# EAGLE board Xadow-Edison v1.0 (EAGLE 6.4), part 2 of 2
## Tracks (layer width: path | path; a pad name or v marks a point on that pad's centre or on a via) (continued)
SPI_MOSI/D11  (via drill 0.1 pad 0.25 layers 1-2, 0.3 pad 0.64) (continued)
  Route2 0.102: v17.14,36.32 17.14,36.96 17.4,37.21 18.16,37.21 18.41,36.96 18.41,36.07 18.16,35.81 18.16,31.75 17.14,30.73 17.14,28.96 18.41,27.69 18.41,25.53 17.53,24.64 17.53,23.88 18.16,23.24 18.16,21.21 20.19,19.18 20.19,17.65 19.56,17.02 19.56,12.95 18.16,11.56 18.16,11.3 18.41,11.05 18.41,10.16 18.16,9.91 18.16,9.27 18.41,9.02 18.41,8.51 18.16,8.26 18.16,6.73 v18.01,6.58
  Bottom 0.102: v10.99,4.7 12.89,4.7 13.91,3.68 13.91,1.97 14.22,1.65 15.11,1.65 15.37,1.91 v15.37,2.29
SYS  (via drill 0.3 pad 0.64)
  Top 0.254: U19.15 v26.42,33.33 v26.42,33.34 | U19.1 25.2,32.21 v25.15,32.26 | v27.56,28.45 27.56,28 R31.1
  Route2 0.61: v25.15,32.26 25.34,32.26 v26.42,33.34
  Bottom 0.254: v25.15,32.26 25.15,28.19 25.65,27.69 26.8,27.69 v27.56,28.45
  Bottom 0.61: v25.15,32.26 24.38,32.26 22.99,30.86 20.45,30.86 19.74,30.15 v19.74,29.62
  pour Top (isolate 0.254, no thermals): 22.22,27.81 21.46,27.81 21.21,28.07 21.21,29.08 20.95,29.34 19.05,29.34 18.8,29.59 18.8,30.61 18.92,30.73 21.84,30.73 21.97,30.61 21.97,29.84 22.1,29.72 22.48,29.72 22.61,29.59 22.61,27.94 22.48,27.81
UART1_CTS  (via drill 0.1 pad 0.25 layers 1-2, 0.3 pad 0.64)
  Top 0.102: U26.4 6.67,10.8 v6.67,10.79 | J2.17 4.08,16.75 v4.06,16.76 | R63.1 v1.46,7.11
  Route2 0.102: v4.06,16.76 4.06,16.38 4.83,15.62 4.83,14.22 4.57,13.97 4.57,13.46 6.67,11.37 v6.67,10.79 6.67,10.48 6.35,10.16 4.06,10.16 1.46,7.56 v1.46,7.11
UART1_RTS  (via drill 0.1 pad 0.25 layers 1-2, 0.3 pad 0.64)
  Top 0.102: U27.4 8.76,8.25 8.38,7.87 v8,7.87 | J2.18 6.47,16.25 6.93,16.71 v7.75,16.71 | R62.1 v1.14,5.33
  Route2 0.102: v7.75,16.71 7.75,16.51 8.95,15.3 9.33,15.3 9.53,15.11 9.53,14.61 8.89,13.97 8.45,13.97 7.81,13.34 7.81,12.08 7.37,11.63 7.37,10.41 6.98,10.03 6.98,8.64 7.75,7.87 v8,7.87 8.26,7.87 8.76,7.37 8.76,5.57 7.39,4.19 2.29,4.19 v1.14,5.33
UART1_RX  (via drill 0.1 pad 0.25 layers 1-2, 0.3 pad 0.64)
  Top 0.102: J3.2 12.88,3.03 v12.83,2.98 | J4.11 12.88,36.04 v12.8,36.12 | U9.4 14.6,10.54 v14.35,10.29 | R59.1 1.84,8.95 2.33,9.44 3.51,9.44 3.94,9.02 v3.94,8.51
  Route2 0.102: v12.83,2.98 12.83,6.1 13.83,7.1 13.83,8.14 13.59,8.38 13.59,9.53 v14.35,10.29 14.48,10.41 14.48,11.81 13.97,12.32 13.97,13.97 13.84,14.1 13.84,18.92 13.34,19.43 13.34,21.72 13.72,22.1 13.97,22.1 14.48,22.61 14.48,23.37 14.26,23.58 14.26,24.68 14.73,25.15 14.73,28.57 15.37,29.21 15.37,30.35 14.86,30.86 13.97,30.86 13.34,31.5 13.34,35.59 v12.8,36.12
  Bottom 0.102: v12.83,2.98 12.19,3.62 10.6,3.62 9.02,2.03 7.11,2.03 4.19,4.95 4.19,8.26 v3.94,8.51 3.94,9.27 P2.00
UART1_TX  (via drill 0.1 pad 0.25 layers 1-2, 0.3 pad 0.64)
  Top 0.102: U8.4 v12.82,10.8 v12.83,10.79 | J3.1 12.38,3.8 v11.62,3.05 | J4.12 12.38,34.1 v12.45,34.04 | R60.1 1.4,8 1.14,8.26 1.14,9.3 v1.52,9.68
  Route2 0.102: v11.62,3.05 11.81,3.24 11.81,7.62 12.08,7.89 12.08,8.88 11.94,9.02 11.94,9.91 v12.83,10.79 12.83,11.68 13.21,12.06 13.21,13.59 13.08,13.72 13.08,18.54 12.57,19.05 12.57,22.61 13.34,23.37 13.34,24.51 14.22,25.4 14.22,28.83 14.86,29.46 14.86,30.1 14.61,30.35 13.72,30.35 12.83,31.24 12.83,33.66 v12.45,34.04
  Bottom 0.102: v1.52,9.68 2.01,9.68 P1.00 2.29,8.51 3.43,7.37 3.43,2.79 4.44,1.78 9.14,1.78 10.41,3.05 v11.62,3.05
USB_DN  (via drill 0.3 pad 0.64)
  Top 0.102: J9.10 26.63,21.43 v26.8,21.27
  Bottom 0.102: J1.18 5.81,19.53 6.73,20.45 7.87,20.45 8.51,19.81 14.99,19.81 15.75,20.57 24,20.57 arc90 24.26,20.83 24.26,20.95 arc-90 24.51,21.21 arc-90 24.77,20.95 24.77,20.83 arc90 25.02,20.57 arc90 25.27,20.83 25.27,20.95 arc-90 25.53,21.21 arc-90 25.78,20.95 25.78,20.83 arc90 26.04,20.57 26.49,20.57 arc45 26.58,20.61 26.76,20.79 arc45 26.8,20.88 v26.8,21.27
USB_DP  (via drill 0.3 pad 0.64)
  Top 0.102: J9.11 26.63,21.93 v26.8,22.1
  Bottom 0.102: J1.16 5.79,19.13 6.86,20.19 7.75,20.19 8.38,19.56 15.11,19.56 15.88,20.32 26.62,20.32 arc45 26.71,20.36 27.3,20.95 arc45 27.34,21.04 27.34,21.5 arc45 27.3,21.59 v26.8,22.1
USB_ID  (via drill 0.3 pad 0.64)
  Top 0.102: J9.3 26.52,17.93 26.96,17.49 26.96,15.91 v26.48,15.43
  Bottom 0.102: J1.3 2.83,16.73 3.05,16.51 3.05,15.62 3.3,15.37 5.21,15.37 5.84,14.73 5.84,14.1 6.22,13.72 10.92,13.72 11.18,13.97 22.61,13.97 22.99,14.35 24.38,14.35 24.77,14.73 24.77,15.62 25.02,15.88 26.04,15.88 v26.48,15.43
USB_VBUS  (via drill 0.3 pad 0.64)
  Top 0.305: J9.8 24.4,20.43 23.88,20.95 23.88,22.92 v23.81,22.99
  Bottom 0.203: J1.20 5.58,19.93 5.59,19.94
  Bottom 0.305: 5.59,19.94 7.37,21.72 14.1,21.72 14.99,22.61 18.99,22.61 19.62,23.24 23.56,23.24 v23.81,22.99
VCC_1V8  (via drill 0.3 pad 0.64)
  Top 0.102: U26.1
  Top 0.203: 27.37,4.25 v27.3,4.32 27.62,4 R39.1
  Top 0.254: U24.1 10.03,12.06 10.03,12.57 | U8.1 11.81,12.19 11.81,12.83 | U9.1 13.72,12.19 13.72,12.7 | U22.1 17.02,12.06 17.02,12.7 | 13.72,12.7 13.72,13.08 | 13.72,12.7 13.97,12.95 | 13.72,12.7 13.46,12.95 | U5.1 18.62,12.37 v18.62,13.16 | U25.1 13.34,8.64 13.34,9.65 | U27.1 v8.26,10.18 | U6.1 18.67,8.89 v18.67,9.65 | U3.1 16.89,8.76 16.89,9.27 | 16.89,9.27 16.89,9.65 | 16.89,9.27 17.14,9.53 | 16.89,9.27 16.64,9.53 | U11.1 14.86,8.89 14.86,9.27 | 14.86,9.27 14.86,9.65 | 14.86,9.27 14.61,9.53 | 14.86,9.27 15.11,9.53 | C4.1 | U26.1 6.1,11.94 v6.1,12.87 | U17.21 v19.43,18.67 19.43,19.3 19.06,19.67 U17.23 | U7.1 11.43,9.86 | 11.43,9.9 11.43,10.18 11.43,10.19 | 11.43,9.86 11.43,9.9 | 11.43,9.9 11.3,10.03 | 11.43,9.86 11.44,9.86 11.61,10.03 | U23.1 8.26,13.01 R47.2 | U10.2 8.99,26.87 v9.14,27.03 | 11.81,12.83 11.81,13.18 | 11.81,12.83 11.56,13.08 | 11.81,12.83 12.07,13.08 | 17.02,12.7 17.02,13.08 | 17.02,12.7 16.76,12.95 | 17.02,12.7 17.27,12.95 | R35.2 v28.96,33.53 | 10.03,12.65 10.03,12.93 | 10.03,12.57 10.03,12.65 | 10.03,12.65 10.31,12.93 | 10.03,12.57 9.78,12.83
  Top 0.305: C4.1 U2.21 | U15.8 12.02,24.25 v11.91,24.14 | U16.8 10.02,34.41 v10.11,34.49 | U14.8 11.8,21.32 v11.56,21.08 | U12.8 11.95,18.53 v11.94,18.54
  Top 0.406: U13.5 v6.24,30.72 5.73,31.23 4.94,31.23 4.57,30.86 4.57,30.23 3.85,29.5 R14.2
  Top 0.508: 16.13,13.08 15.49,13.08 | 15.49,13.08 13.72,13.08 12.8,13.08 v12.7,13.18 | v18.67,9.65 16.89,9.65 14.86,9.65 13.34,9.65 12.8,10.19 11.43,10.19 9.78,10.19 | v8.26,10.18 v8.26,10.19 9.78,10.19 | C4.1 C3.1 14.99,23.75 15.27,24.03 v15.32,24.03 | R46.2 15.88,12.7 | 15.88,12.7 15.88,12.83 16.13,13.08 | 15.88,12.7 15.49,13.08 | R30.2 10.08,9.88 | 10.08,9.88 9.78,10.19 | 10.08,9.88 10.34,10.13 | R42.2 12.83,13.31 v12.7,13.18 | R36.2 7.05,38.16 7.05,37.96 v6.86,37.77 6.78,37.85 Q4.1 | Q3.1 6.1,35.56 6.54,36.01 R2.2 | R15.1 v11.15,26.29 | 11.02,13.18 Q2.1 | v12.7,13.18 11.81,13.18 11.02,13.18 | 16.13,13.08 17.02,13.08 17.14,13.08 17.21,13.14 17.27,13.21 Q1.1 | C14.1 9.42,27.3 v9.14,27.03 | R40.2 18.41,13.41 18.67,13.16 18.54,13.16 | R47.2 9.27,13.08 9.42,12.93 v9.53,12.93 10.03,12.93 10.13,12.93 10.39,13.18 11.02,13.18
  Top 0.61: v19.43,18.67 19.88,18.67 C17.1 | v10.11,34.49 10.11,34.85 9.78,35.18 8.38,35.18 8.13,35.43 | 8.13,35.43 v8.13,35.37 | v18.62,13.16 18.54,13.16 17.22,13.16 17.21,13.14 | R2.2 7.56,36.01 8.13,35.43 | v7.19,19.1 7.3,19.21 C33.1 C34.1
  Route2 0.203: v22.99,38.73 22.73,38.73 22.61,38.61
  Route2 0.61: v12.7,13.18 12.57,13.31 12.57,17.91 v11.94,18.54 11.94,20.7 v11.56,21.08 | v15.32,24.03 15.6,24.03 17.4,22.23 17.4,20.7 v19.43,18.67 19.43,18.03 18.62,17.22 v18.62,13.16 | v8.13,35.37 8.13,38.23 | 8.51,38.61 7.75,38.61 | 8.13,38.23 7.75,38.61 | 8.13,38.23 8.51,38.61 | v6.24,30.72 7.05,31.53 8.47,31.53 9.91,30.1 9.91,29.34 9.4,28.83 9.4,27.28 v9.14,27.03 | v6.86,37.77 6.86,38.23 7.24,38.61 7.75,38.61 | v28.96,33.53 27.56,34.92 27.56,35.69 24.64,38.61 22.61,38.61 8.51,38.61
  Bottom 0.203: J1.12 6.81,18.33 | 6.81,18.33 7.41,18.33 7.46,18.38 | v27.3,4.32 27.81,4.32 28.32,4.83 28.32,5.71 28.83,6.22 28.83,9.14 28.45,9.53 28.45,10.92 29.63,12.11 29.63,16.21 28.51,17.34 26.8,17.34 25.53,18.61 19.49,18.61 v19.43,18.67 | 6.81,18.33 6.81,18.37 7.11,18.67 | 1.8V.T v22.99,38.73
  Bottom 0.508: 9.17,27.05 v9.14,27.03 | v6.1,12.87 6.13,12.87 6.22,12.95 9.5,12.95 v9.53,12.93
  Bottom 0.61: v18.67,9.65 18.67,10.03 20.57,11.94 20.57,12.7 20.12,13.16 v18.62,13.16 | v15.32,24.03 13.08,24.03 | 13.08,24.03 12.57,24.03 | 12.57,24.03 12.03,24.03 v11.91,24.14 | 13.08,24.64 13.08,24.51 | 13.08,24.51 13.08,24.03 | 13.08,24.51 13.06,24.51 12.57,24.03 | 13.08,24.64 13.59,24.13 | v8.13,35.37 8.06,35.37 6.73,34.04 6.73,31.21 v6.24,30.72 | 13.08,24.64 13.08,25.53 12.32,26.29 v11.15,26.29 9.88,26.29 v9.14,27.03 | v7.19,19.1 7.19,18.66 7.46,18.38 7.75,18.1 11.49,18.1 v11.94,18.54
VCC_3V3  (via drill 0.3 pad 0.64)
  Top 0.203: R38.1 27.88,6.22 v28.19,6.54
  Top 0.254: U7.6 v12.41,9.39 v12.42,9.4 | U11.6 v15.87,8.89 v15.88,8.89 | U3.6 v17.78,8.89 | U25.6 v14.09,8.89 v14.1,8.89 | U24.6 v10.79,12.31 v10.79,12.32 | U22.6 v17.78,12.31 v17.78,12.32 | U27.6 9.17,9.52 v9.24,9.45 | U18.21 6.47,8.01 v6.1,8.38 | U9.6 14.6,12.19 v14.73,12.31 | U8.6 v12.7,12.31 v12.7,12.32 | U5.6 v19.68,12.26 v19.68,12.27 | U6.6 19.68,8.77 v19.56,8.89 | U18.18 v8.22,7.23 v8.23,7.24 | U4.21 21.97,10.03 21.78,9.84 C16.1 | U26.6 v6.73,12.21 v6.73,12.22 | U23.6 8.76,11.93 v9.02,12.19
  Top 0.305: J3.5 14.38,4.04 14.68,3.73 v15.27,3.73 15.54,3.73 15.88,4.07 J3.8 | v6.71,17.6 6.48,17.83 6.48,18.92 6.15,19.25 J2.12 | 15.62,33.78 14.61,33.78 14.38,34.01 J4.8 14.38,36.22 v15.11,36.96 | 15.62,33.78 15.88,33.78 | 15.88,33.78 16.13,33.78 | 16.13,33.78 v19.18,33.78 | 15.88,33.78 | J4.5 15.88,34.03 | 15.88,34.03 16.13,33.78 | 15.88,34.03 15.87,34.03 15.62,33.78
  Top 0.508: R41.2 13.97,14.92 v14.35,15.3 | C16.1 21.21,9.35 v21.18,9.32 21.21,9.3 R44.2 | R67.2 R3.2 3.87,37.02 v3.94,37.08 | C7.1 20.07,22.73 v19.84,22.5 19.46,22.5 19.18,22.23 R7.2
  Top 0.61: C32.1 C31.1 7.04,17.27 v6.71,17.6 | R43.2 6.6,14.1 v6.41,14.29 | v19.68,12.26 19.68,12.66 20.99,13.97 21.84,13.97 22.29,14.41 R45.2 22.73,14.99 v22.48,15.24
  Route2 0.203: v28.19,6.54 28.19,9.98 26.49,11.68 23.88,11.68 23.43,12.13 23.43,14.29 v22.48,15.24
  Route2 0.508: v14.35,15.3 14.35,14.73 14.73,14.35 v14.73,12.31 | v15.11,36.96 15.11,37.08 14.5,37.7 11.54,37.7 v10.16,36.32
  Route2 0.61: v6.71,17.6 6.35,17.25 6.35,14.35 v6.41,14.29 6.86,13.84 6.86,12.34 v6.73,12.22 | v19.56,8.89 20.07,8.89 20.5,9.32 v21.18,9.32 | v19.18,33.78 19.18,31.24 18.92,30.99 18.92,29.08 19.68,28.32 19.68,22.66 v19.84,22.5 23.38,18.96 23.38,17.04 22.48,16.13 v22.48,15.24
  Bottom 0.203: J1.8 6.63,17.53 v6.71,17.6 6.38,17.93 J1.10 | 3.3V.T 16.89,38.73 v15.11,36.96
  Bottom 0.508: v14.1,8.89 v15.88,8.89 v17.78,8.89 v19.56,8.89 | v14.73,12.31 v17.78,12.31 v17.78,12.32 19.63,12.32 v19.68,12.27 | v10.79,12.32 v12.7,12.32 v14.72,12.32 v14.73,12.31 | v9.24,9.45 9.24,9.5 9.65,9.91 11.91,9.91 v12.42,9.4 13.59,9.4 v14.1,8.89 | v14.73,12.32 v14.73,12.31 | v14.1,8.89 14.1,5.46 15.24,4.32 15.24,3.76 v15.27,3.73 | 6.76,17.65 v6.71,17.6 | v8.23,7.24 7.09,8.38 v6.1,8.38
  Bottom 0.61: v9.24,9.45 9.24,7.72 8.76,7.24 v8.23,7.24 | v17.78,8.89 v17.78,12.32 | v3.94,37.08 4.62,36.4 10.08,36.4 v10.16,36.32 | v10.79,12.32 10.79,12.29 10.59,12.09 9.12,12.09 v9.02,12.19 8.99,12.22 v6.73,12.22
VCC_4V3  (via drill 0.3 pad 0.64)
  Top 0.305: U28.7 22.35,17.91 v22.54,17.72 | U28.8 22.85,17.89 22.67,17.72 | U28.5 21.35,17.82 v21.25,17.72
  Top 0.61: R33.1 19.43,31.42 19.46,31.42 v19.94,31.9 | v23.94,15.43 C24.1 C23.1 R24.1 22.92,17.46 22.67,17.72 v22.54,17.72
  Route2 0.203: v27.3,17.91 25.65,17.91 | 25.65,17.91 25.27,17.91 | 25.65,17.91 25.4,18.16 25.4,17.65 25.65,17.91
  Route2 0.61: v19.94,31.9 21.46,30.38 21.46,22.35 25.27,18.54 25.27,17.91 25.27,16.26 24.45,15.43 v23.94,15.43
  Bottom 0.203: v27.3,17.91 28.19,17.91 4.3V.T
  Bottom 0.61: v22.54,17.72 v21.25,17.72
VCC_SDIO  (via drill 0.1 pad 0.25 layers 1-2)
  Top 0.254: U10.7 | J2.9 5.98,20.75 6.25,21.02 6.25,21.29 6.73,21.77 7.92,21.77 v8.13,21.97
  Route2 0.254: U10.7 8.48,26.47 9.14,25.8 9.14,24.38 8.13,23.37 v8.13,21.97
  other vias: 7.77,26.47
VCC_SYS  (via drill 0.1 pad 0.25 layers 1-2, 0.3 pad 0.64)
  Top 0.203: C29.1 6.35,15.11 5.84,14.61 5.21,14.61 4.57,13.97 | v27.18,24.45 C22.1 27.24,25.08 28.19,26.04 R70.1
  Top 0.254: U10.6
  Top 0.508: v8.08,28.35 8.08,28.82 C15.1 | v27.56,16.64 27.56,13.65 R32.1
  Top 0.61: C30.1 7.3,15.76 v7.29,15.75 7.3,15.73 C29.1 | R26.1 22.41,23.81 L2.2 22.99,24 22.99,24.77 23.3,25.08 23.37,25.08 | v25.08,26.1 C6.1 R37.1 23.37,25.08 | C22.1 C21.1 C19.1 C20.1 23.37,25.08
  Route2 0.254: U10.6 7.77,27.58 8.08,27.89 v8.08,28.35
  Route2 0.61: v27.56,16.64 28.19,17.27 28.19,18.54 25.91,20.83 25.91,25.27 v25.08,26.1
  Bottom 0.203: J1.4 6.26,16.73 | 6.26,16.73 6.38,16.73 | J1.6 6.24,17.13 6.38,16.98 6.38,16.82 | 6.38,16.73 6.38,16.82 | 6.38,16.82 6.3,16.74 | 6.38,16.73 6.38,16.09 | 6.38,16.09 6.73,15.75 v7.29,15.75 | 6.26,16.73 6.35,16.64 | J1.2 6.15,16.33 | 6.15,16.33 6.38,16.09 | 6.15,16.33 6.27,16.33 6.38,16.43 | v27.18,24.45 28.38,24.45 VSYS.T
  Bottom 0.61: v8.08,28.35 8.69,28.96 9.53,28.96 11.18,30.61 15.37,30.61 16.81,29.16 18.59,29.16 19.94,27.81 22.48,27.81 24.19,26.1 v25.08,26.1 | v7.29,15.75 7.3,15.75 8.83,17.27 12.7,17.27 13.72,18.29 14.73,18.29 16.13,16.89 23.11,16.89 24.13,17.91 25.15,17.91 26.42,16.64 v27.56,16.64
  other vias: 7.77,26.87
  pour Top (isolate 0.254, no thermals): 22.99,26.29 25.53,26.29 25.53,24.89 22.99,24.89
VCC_USB  (via drill 0.3 pad 0.64, 0.3 pad 0.64 layers 1-2)
  Top 0.305: U19.2 23.56,31.11 C26.2 | J9.5 26.66,18.93 26.8,18.8 v26.8,18.67 26.56,18.43 J9.4
  Top 0.61: C26.2 C25.2 v22.48,31.88
  Route2 0.61: v22.48,31.88 22.48,27.5 24.89,25.08 24.89,20.57 v26.8,18.67
WP/CD  (via drill 0.1 pad 0.25 layers 1-2)
  Top 0.102: R23.1 R15.2 9.65,26.29 9.02,25.65 v8.64,25.65 8.64,26.16 8.33,26.47 U10.3 | J2.7 6,21.75 v6.22,21.97
  Route2 0.102: v8.64,25.65 8.64,24.38 v6.22,21.97

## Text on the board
tPlace: 1 | - | + | 1 | 1 | 1
bPlace: Xadow | Xadow-Edison | v1.0 10/29/2014 | by Seeed Studio | www.seeedstudio.com | Programmer | Xadow
bNames: D7 | D8 | UART1_TX | UART1_RX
